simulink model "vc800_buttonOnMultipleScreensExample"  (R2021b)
settings: Solver=FixedStepDiscrete  StartTime=0.0  StopTime=10.0  FixedStep=0.01  RelTol=1e-3  EnableMultiTasking=on
PreLoadFcn:
  | try, model_open; catch, disp('Error occurred while executing model pre-load callback: model_open.m'); disp('Please assure that the MATLAB working directory is set to the model directory before opening.'); end
InitFcn:
  | try, model_open; catch, end
model workspace (MAT data in the model file):
  IOScreen_Label_XCoord = 1
  IOScreen_Row1_YCoord = 1
  IOScreen_Row2_YCoord = 12
  IOScreen_Value_XCoord = 110
  MainScreen_Row1_YCoord = 7
  MainScreen_Row2_YCoord = 23
  MainScreen_Symbols_XCoord = 1
  MainScreen_Units_XCoord = 69
  MainScreen_Value_XCoord = 64
undefined symbols (not defined in the file or in its folder): case, curr_screen, default, DISP, filtering, gesture, hex2dec, Mode, No, raptor_get_buildNum, raptor_get_safe_string, raptor_hwexp, raptor_xcp_function, Screens, VC800, Voltage
libraries: Raptor_display_lib x190, Raptor_lib x97, simulink_extras x11, Raptor_Datalogging_lib x10, simulink x2
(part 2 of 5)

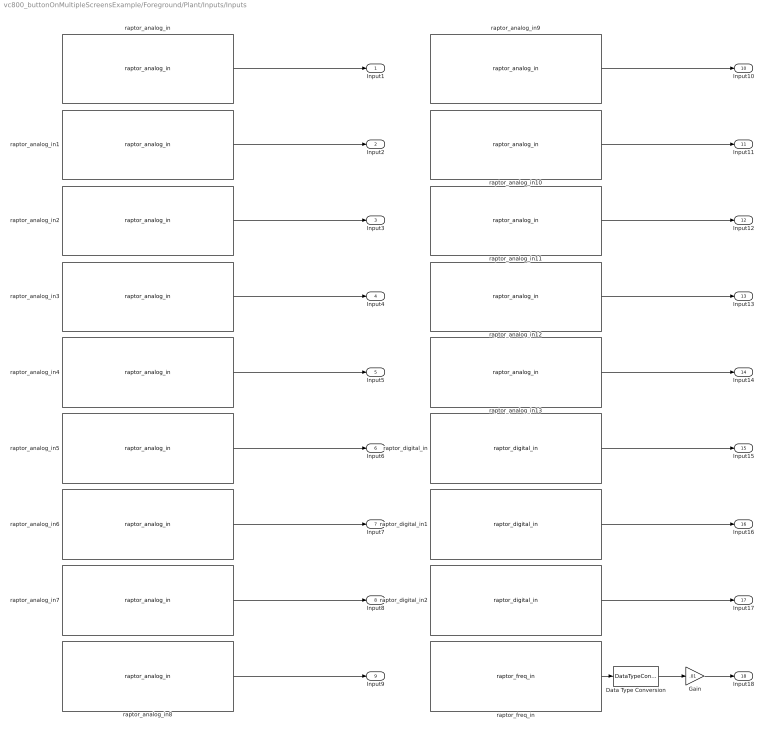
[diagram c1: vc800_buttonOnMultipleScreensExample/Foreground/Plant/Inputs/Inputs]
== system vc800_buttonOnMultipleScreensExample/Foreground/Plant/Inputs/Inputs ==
  Data Type Conversion : DataTypeConversion  OutDataTypeStr=single
  Gain : Gain  Gain=.01
  raptor_analog_in : Raptor_lib/Input & Output/raptor_analog_in  resourceValues=INPUT1|INPUT2|INPUT3|INPUT4|INPUT5|INPUT6|INPUT7|INPUT8|INPUT9|INPUT10|INPUT11|INPUT12|INPUT13|INPUT14|(None)  resource=INPUT1  rangeValues=Voltage Mode (0-10V)|Resistance Mode (0-500 Ohms)  range=Voltage Mode (0-10V)  filterrateValues=0.01 (~10 sec)|0.02|0.05|0.10 (Default)|0.25|0.50|0.75|1.00 (No filtering)  filterrate=1.00 (No filtering)  resolutionValues=[]  resolution=[]  pullUDValues=[]  pullUD=[]
  raptor_analog_in1 : Raptor_lib/Input & Output/raptor_analog_in  resourceValues=INPUT1|INPUT2|INPUT3|INPUT4|INPUT5|INPUT6|INPUT7|INPUT8|INPUT9|INPUT10|INPUT11|INPUT12|INPUT13|INPUT14|(None)  resource=INPUT2  rangeValues=Voltage Mode (0-10V)|Resistance Mode (0-500 Ohms)  range=Voltage Mode (0-10V)  filterrateValues=0.01 (~10 sec)|0.02|0.05|0.10 (Default)|0.25|0.50|0.75|1.00 (No filtering)  filterrate=1.00 (No filtering)  resolutionValues=[]  resolution=[]  pullUDValues=[]  pullUD=[]
  raptor_analog_in10 : Raptor_lib/Input & Output/raptor_analog_in  resourceValues=INPUT1|INPUT2|INPUT3|INPUT4|INPUT5|INPUT6|INPUT7|INPUT8|INPUT9|INPUT10|INPUT11|INPUT12|INPUT13|INPUT14|(None)  resource=INPUT11  rangeValues=Voltage Mode (0-10V)|Resistance Mode (0-500 Ohms)  range=Voltage Mode (0-10V)  filterrateValues=0.01 (~10 sec)|0.02|0.05|0.10 (Default)|0.25|0.50|0.75|1.00 (No filtering)  filterrate=1.00 (No filtering)  resolutionValues=[]  resolution=[]  pullUDValues=[]  pullUD=[]
  raptor_analog_in11 : Raptor_lib/Input & Output/raptor_analog_in  resourceValues=INPUT1|INPUT2|INPUT3|INPUT4|INPUT5|INPUT6|INPUT7|INPUT8|INPUT9|INPUT10|INPUT11|INPUT12|INPUT13|INPUT14|(None)  resource=INPUT12  rangeValues=Voltage Mode (0-10V)|Resistance Mode (0-500 Ohms)  range=Voltage Mode (0-10V)  filterrateValues=0.01 (~10 sec)|0.02|0.05|0.10 (Default)|0.25|0.50|0.75|1.00 (No filtering)  filterrate=1.00 (No filtering)  resolutionValues=[]  resolution=[]  pullUDValues=[]  pullUD=[]
  raptor_analog_in12 : Raptor_lib/Input & Output/raptor_analog_in  resourceValues=INPUT1|INPUT2|INPUT3|INPUT4|INPUT5|INPUT6|INPUT7|INPUT8|INPUT9|INPUT10|INPUT11|INPUT12|INPUT13|INPUT14|(None)  resource=INPUT13  rangeValues=Voltage Mode (0-10V)|Resistance Mode (0-500 Ohms)  range=Voltage Mode (0-10V)  filterrateValues=0.01 (~10 sec)|0.02|0.05|0.10 (Default)|0.25|0.50|0.75|1.00 (No filtering)  filterrate=1.00 (No filtering)  resolutionValues=[]  resolution=[]  pullUDValues=[]  pullUD=[]
  raptor_analog_in13 : Raptor_lib/Input & Output/raptor_analog_in  resourceValues=INPUT1|INPUT2|INPUT3|INPUT4|INPUT5|INPUT6|INPUT7|INPUT8|INPUT9|INPUT10|INPUT11|INPUT12|INPUT13|INPUT14|(None)  resource=INPUT14  rangeValues=Voltage Mode (0-10V)|Resistance Mode (0-500 Ohms)  range=Voltage Mode (0-10V)  filterrateValues=0.01 (~10 sec)|0.02|0.05|0.10 (Default)|0.25|0.50|0.75|1.00 (No filtering)  filterrate=1.00 (No filtering)  resolutionValues=[]  resolution=[]  pullUDValues=[]  pullUD=[]
  raptor_analog_in2 : Raptor_lib/Input & Output/raptor_analog_in  resourceValues=INPUT1|INPUT2|INPUT3|INPUT4|INPUT5|INPUT6|INPUT7|INPUT8|INPUT9|INPUT10|INPUT11|INPUT12|INPUT13|INPUT14|(None)  resource=INPUT3  rangeValues=Voltage Mode (0-10V)|Resistance Mode (0-500 Ohms)  range=Voltage Mode (0-10V)  filterrateValues=0.01 (~10 sec)|0.02|0.05|0.10 (Default)|0.25|0.50|0.75|1.00 (No filtering)  filterrate=1.00 (No filtering)  resolutionValues=[]  resolution=[]  pullUDValues=[]  pullUD=[]
  raptor_analog_in3 : Raptor_lib/Input & Output/raptor_analog_in  resourceValues=INPUT1|INPUT2|INPUT3|INPUT4|INPUT5|INPUT6|INPUT7|INPUT8|INPUT9|INPUT10|INPUT11|INPUT12|INPUT13|INPUT14|(None)  resource=INPUT4  rangeValues=Voltage Mode (0-10V)|Resistance Mode (0-500 Ohms)  range=Voltage Mode (0-10V)  filterrateValues=0.01 (~10 sec)|0.02|0.05|0.10 (Default)|0.25|0.50|0.75|1.00 (No filtering)  filterrate=1.00 (No filtering)  resolutionValues=[]  resolution=[]  pullUDValues=[]  pullUD=[]
  raptor_analog_in4 : Raptor_lib/Input & Output/raptor_analog_in  resourceValues=INPUT1|INPUT2|INPUT3|INPUT4|INPUT5|INPUT6|INPUT7|INPUT8|INPUT9|INPUT10|INPUT11|INPUT12|INPUT13|INPUT14|(None)  resource=INPUT5  rangeValues=Voltage Mode (0-10V)|Resistance Mode (0-500 Ohms)  range=Voltage Mode (0-10V)  filterrateValues=0.01 (~10 sec)|0.02|0.05|0.10 (Default)|0.25|0.50|0.75|1.00 (No filtering)  filterrate=1.00 (No filtering)  resolutionValues=[]  resolution=[]  pullUDValues=[]  pullUD=[]
  raptor_analog_in5 : Raptor_lib/Input & Output/raptor_analog_in  resourceValues=INPUT1|INPUT2|INPUT3|INPUT4|INPUT5|INPUT6|INPUT7|INPUT8|INPUT9|INPUT10|INPUT11|INPUT12|INPUT13|INPUT14|(None)  resource=INPUT6  rangeValues=Voltage Mode (0-10V)|Resistance Mode (0-500 Ohms)  range=Voltage Mode (0-10V)  filterrateValues=0.01 (~10 sec)|0.02|0.05|0.10 (Default)|0.25|0.50|0.75|1.00 (No filtering)  filterrate=1.00 (No filtering)  resolutionValues=[]  resolution=[]  pullUDValues=[]  pullUD=[]
  raptor_analog_in6 : Raptor_lib/Input & Output/raptor_analog_in  resourceValues=INPUT1|INPUT2|INPUT3|INPUT4|INPUT5|INPUT6|INPUT7|INPUT8|INPUT9|INPUT10|INPUT11|INPUT12|INPUT13|INPUT14|(None)  resource=INPUT7  rangeValues=Voltage Mode (0-10V)|Resistance Mode (0-500 Ohms)  range=Voltage Mode (0-10V)  filterrateValues=0.01 (~10 sec)|0.02|0.05|0.10 (Default)|0.25|0.50|0.75|1.00 (No filtering)  filterrate=1.00 (No filtering)  resolutionValues=[]  resolution=[]  pullUDValues=[]  pullUD=[]
  raptor_analog_in7 : Raptor_lib/Input & Output/raptor_analog_in  resourceValues=INPUT1|INPUT2|INPUT3|INPUT4|INPUT5|INPUT6|INPUT7|INPUT8|INPUT9|INPUT10|INPUT11|INPUT12|INPUT13|INPUT14|(None)  resource=INPUT8  rangeValues=Voltage Mode (0-10V)|Resistance Mode (0-500 Ohms)  range=Voltage Mode (0-10V)  filterrateValues=0.01 (~10 sec)|0.02|0.05|0.10 (Default)|0.25|0.50|0.75|1.00 (No filtering)  filterrate=1.00 (No filtering)  resolutionValues=[]  resolution=[]  pullUDValues=[]  pullUD=[]
  raptor_analog_in8 : Raptor_lib/Input & Output/raptor_analog_in  resourceValues=INPUT1|INPUT2|INPUT3|INPUT4|INPUT5|INPUT6|INPUT7|INPUT8|INPUT9|INPUT10|INPUT11|INPUT12|INPUT13|INPUT14|(None)  resource=INPUT9  rangeValues=Voltage Mode (0-10V)|Resistance Mode (0-500 Ohms)  range=Voltage Mode (0-10V)  filterrateValues=0.01 (~10 sec)|0.02|0.05|0.10 (Default)|0.25|0.50|0.75|1.00 (No filtering)  filterrate=1.00 (No filtering)  resolutionValues=[]  resolution=[]  pullUDValues=[]  pullUD=[]
  raptor_analog_in9 : Raptor_lib/Input & Output/raptor_analog_in  resourceValues=INPUT1|INPUT2|INPUT3|INPUT4|INPUT5|INPUT6|INPUT7|INPUT8|INPUT9|INPUT10|INPUT11|INPUT12|INPUT13|INPUT14|(None)  resource=INPUT10  rangeValues=Voltage Mode (0-10V)|Resistance Mode (0-500 Ohms)  range=Voltage Mode (0-10V)  filterrateValues=0.01 (~10 sec)|0.02|0.05|0.10 (Default)|0.25|0.50|0.75|1.00 (No filtering)  filterrate=1.00 (No filtering)  resolutionValues=[]  resolution=[]  pullUDValues=[]  pullUD=[]
  raptor_digital_in : Raptor_lib/Input & Output/raptor_digital_in  resourceValues=INPUT15|INPUT16|INPUT17|(None)  resource=INPUT15  pullUDValues=[]  pullUD=[]  upperThres='RAPTOR MASK DEFAULT'  lowerThres='RAPTOR MASK DEFAULT'
  raptor_digital_in1 : Raptor_lib/Input & Output/raptor_digital_in  resourceValues=INPUT15|INPUT16|INPUT17|(None)  resource=INPUT16  pullUDValues=[]  pullUD=[]  upperThres='RAPTOR MASK DEFAULT'  lowerThres='RAPTOR MASK DEFAULT'
  raptor_digital_in2 : Raptor_lib/Input & Output/raptor_digital_in  resourceValues=INPUT15|INPUT16|INPUT17|(None)  resource=INPUT17  pullUDValues=[]  pullUD=[]  upperThres='RAPTOR MASK DEFAULT'  lowerThres='RAPTOR MASK DEFAULT'
  raptor_freq_in : Raptor_lib/Input & Output/raptor_freq_in  minFreq=1  resourceValues=INPUT18|(None)  resource=INPUT18  pullUDValues=[]  pullUD=[]  interfaceValues=[]  interface=[]  hasDuty='RAPTOR MASK DEFAULT'  hasEdgeCount=off
  Input1 : Outport  VectorParamsAs1DForOutWhenUnconnected=off
  Input2 : Outport  Port=2  VectorParamsAs1DForOutWhenUnconnected=off
  Input3 : Outport  Port=3  VectorParamsAs1DForOutWhenUnconnected=off
  Input4 : Outport  Port=4  VectorParamsAs1DForOutWhenUnconnected=off
  Input5 : Outport  Port=5  VectorParamsAs1DForOutWhenUnconnected=off
  Input6 : Outport  Port=6  VectorParamsAs1DForOutWhenUnconnected=off
  Input7 : Outport  Port=7  VectorParamsAs1DForOutWhenUnconnected=off
  Input8 : Outport  Port=8  VectorParamsAs1DForOutWhenUnconnected=off
  Input9 : Outport  Port=9  VectorParamsAs1DForOutWhenUnconnected=off
  Input10 : Outport  Port=10  VectorParamsAs1DForOutWhenUnconnected=off
  Input11 : Outport  Port=11  VectorParamsAs1DForOutWhenUnconnected=off
  Input12 : Outport  Port=12  VectorParamsAs1DForOutWhenUnconnected=off
  Input13 : Outport  Port=13  VectorParamsAs1DForOutWhenUnconnected=off
  Input14 : Outport  Port=14  VectorParamsAs1DForOutWhenUnconnected=off
  Input15 : Outport  Port=15  VectorParamsAs1DForOutWhenUnconnected=off
  Input16 : Outport  Port=16  VectorParamsAs1DForOutWhenUnconnected=off
  Input17 : Outport  Port=17  VectorParamsAs1DForOutWhenUnconnected=off
  Input18 : Outport  Port=18  VectorParamsAs1DForOutWhenUnconnected=off
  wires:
  raptor_analog_in/1 -> Input1/1
  raptor_analog_in1/1 -> Input2/1
  raptor_analog_in2/1 -> Input3/1
  raptor_analog_in3/1 -> Input4/1
  raptor_analog_in4/1 -> Input5/1
  raptor_analog_in9/1 -> Input10/1
  raptor_analog_in8/1 -> Input9/1
  raptor_analog_in7/1 -> Input8/1
  raptor_analog_in6/1 -> Input7/1
  raptor_analog_in5/1 -> Input6/1
  raptor_analog_in12/1 -> Input13/1
  raptor_analog_in13/1 -> Input14/1
  raptor_analog_in11/1 -> Input12/1
  raptor_analog_in10/1 -> Input11/1
  raptor_digital_in/1 -> Input15/1
  raptor_digital_in2/1 -> Input17/1
  raptor_digital_in1/1 -> Input16/1
  raptor_freq_in/1 -> Data Type Conversion/1
  Gain/1 -> Input18/1
  Data Type Conversion/1 -> Gain/1

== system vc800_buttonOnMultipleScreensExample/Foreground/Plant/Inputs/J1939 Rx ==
  Process Illumination Message : Subsystem
  Process RPM Message : Subsystem
  raptor_can_rxmsg : Raptor_lib/CAN/raptor_can_rxmsg  canDefinition="struct('dbcFile', 'j1939_small.dbc','message', 'CL','comment', '','signals', {{'IlluminationBrightnessPercent'}},'enabled', [ 1;],'canBus', '''CAN1''','messageID', [ 416349696;],'idMask', [ 536870656;],'payloadMask', [],'payloadValue', [],'period', [ 0;],'mailbox', '''''','queueSize', [ 1;],'label', [ 0;],'ver', [ 2;],'showID', [ 0;],'showRaw', [ 0;],'fill', [ 0;],'editID', [ 1;],'signalOrder', [ 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"  canBus='CAN1'  mailbox=''  payloadMask=[]  payloadValue=[]  idMask=hex2dec('1FFFFF00')  queueSize=1  showID=0  label=0  fill=0  id=416349696  showRaw=0  showAge=1  signalOrder=1  signalInfo={{struct('Name', 'IlluminationBrightnessPercent','StartBit', [ 0;],'SignalSize', [ 8;],'ByteOrder', 'LittleEndian','ValueType', 'UNSIGNED','Class', 'uint8','Signed', [ 0;],'Factor', [ 0.4;],'Offset', [ 0;],'Min', [ 0;],'Max', [ 100;],'Units', '%','StartVal', [ 0;],'Comment', 'Commanded backlight brightness level for all cab displays','Multiplexed', [ 0;],'Multiplexor', [ 0;],'MultiplexMode_Min', [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  showRawMsg=0  useSimFunc=0  sim_func_name=''  useStartVals=0  extendedId=1
  raptor_can_rxmsg1 : Raptor_lib/CAN/raptor_can_rxmsg  canDefinition=struct('dbcFile', 'j1939_small.dbc','message', 'EEC1','comment', '','signals', {{'EngSpeed'}},'enabled', [ 1;],'canBus', '''CAN1''','messageID', [ 217056256;],'idMask', [ 536870656;],'payloadMask', [],'payloadValue', [],'period', [ 0;],'mailbox', '''''','queueSize', [ 1;],'label', [ 0;],'ver', [ 2;],'showID', [ 0;],'showRaw', [ 0;],'fill', [ 0;],'editID', [ 1;],'signalOrder', [ 1;])  canBus='CAN1'  mailbox=''  payloadMask=[]  payloadValue=[]  idMask=hex2dec('1FFFFF00')  queueSize=1  showID=0  label=0  fill=0  id=217056256  showRaw=0  showAge=1  signalOrder=1  signalInfo={{struct('Name', 'EngSpeed','StartBit', [ 24;],'SignalSize', [ 16;],'ByteOrder', 'LittleEndian','ValueType', 'UNSIGNED','Class', 'uint16','Signed', [ 0;],'Factor', [ 0.125;],'Offset', [ 0;],'Min', [ 0;],'Max', [ 8031.88;],'Units', 'rpm','StartVal', [ 0;],'Comment', 'Actual engine speed which is calculated over a minimum crankshaft angle of 720 degrees divided by the number of cylinders.','Multiple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  showRawMsg=0  useSimFunc=0  sim_func_name=''  useStartVals=0  extendedId=1
  Engine RPM : Outport  VectorParamsAs1DForOutWhenUnconnected=off
  Engine RPM Valid : Outport  Port=2  VectorParamsAs1DForOutWhenUnconnected=off
  Illumination : Outport  Port=3  VectorParamsAs1DForOutWhenUnconnected=off
  Illumination1 : Outport  Port=4  VectorParamsAs1DForOutWhenUnconnected=off
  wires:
  Process RPM Message/1(EngineRPM) -> Engine RPM/1
  Process Illumination Message/1(Illumination) -> Illumination/1
  Process RPM Message/2(EngineRPMValid) -> Engine RPM Valid/1
  raptor_can_rxmsg1/1 -> Process RPM Message/1(AgeCount)
  raptor_can_rxmsg1/2 -> Process RPM Message/2(Data)
  raptor_can_rxmsg/1 -> Process Illumination Message/1(AgeCount)
  raptor_can_rxmsg/2 -> Process Illumination Message/2(Data)
  Process Illumination Message/2(IlluminationValid) -> Illumination1/1

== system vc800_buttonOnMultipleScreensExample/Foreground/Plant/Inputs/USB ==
  raptor_fileIO_USBStatus : Raptor_Datalogging_lib/raptor_fileIO_USBStatus  showInserted=on  showEjectReady=on  showPath=on  showReadyToLog=on
  raptor_fileIO_getFreeSpace : Raptor_Datalogging_lib/raptor_fileIO_getFreeSpace  resourceValues=USB|(None)  resource=USB
  raptor_string : Raptor_lib/Strings/raptor_string  stringName=''  string=''  dynamicSize=Fixed Size  strSize=20  storage=Volatile (RAM)  calVisible=off  calAccess=4  strFunction=raptor_xcp_function(gcb)
  USBInserted : Outport  VectorParamsAs1DForOutWhenUnconnected=off
  USBEjectReady : Outport  Port=2  VectorParamsAs1DForOutWhenUnconnected=off
  USBPath : Outport  Port=3  VectorParamsAs1DForOutWhenUnconnected=off
  USBReadyToLog : Outport  Port=4  VectorParamsAs1DForOutWhenUnconnected=off
  USBFreeSpace : Outport  Port=5  VectorParamsAs1DForOutWhenUnconnected=off
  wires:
  raptor_fileIO_USBStatus/1 -> USBInserted/1
  raptor_fileIO_USBStatus/4 -> USBReadyToLog/1
  raptor_fileIO_USBStatus/3 -> USBPath/1
  raptor_fileIO_USBStatus/2 -> USBEjectReady/1
  raptor_string/1 -> raptor_fileIO_USBStatus/1
  raptor_fileIO_getFreeSpace/1 -> USBFreeSpace/1

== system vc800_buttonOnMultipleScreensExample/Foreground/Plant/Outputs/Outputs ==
  Output1 : Inport
  Output2 : Inport  Port=2
  Output3 : Inport  Port=3
  Output4 : Inport  Port=4
  Output5 : Inport  Port=5
  Output6 : Inport  Port=6
  Output7 : Inport  Port=7
  Output8 : Inport  Port=8
  raptor_digital_out : Raptor_lib/Input & Output/raptor_digital_out  resourceValues=OUTPUT1|OUTPUT2|OUTPUT3|OUTPUT4|BUZZER_MUTE|BUZZER|OUTPUT5|OUTPUT6|OUTPUT7|OUTPUT8|(None)  resource=OUTPUT1  driverTypeValues=Low Side  driverType=Low Side
  raptor_digital_out1 : Raptor_lib/Input & Output/raptor_digital_out  resourceValues=OUTPUT1|OUTPUT2|OUTPUT3|OUTPUT4|BUZZER_MUTE|BUZZER|OUTPUT5|OUTPUT6|OUTPUT7|OUTPUT8|(None)  resource=OUTPUT2  driverTypeValues=Low Side  driverType=Low Side
  raptor_digital_out2 : Raptor_lib/Input & Output/raptor_digital_out  resourceValues=OUTPUT1|OUTPUT2|OUTPUT3|OUTPUT4|BUZZER_MUTE|BUZZER|OUTPUT5|OUTPUT6|OUTPUT7|OUTPUT8|(None)  resource=OUTPUT3  driverTypeValues=Low Side  driverType=Low Side
  raptor_digital_out3 : Raptor_lib/Input & Output/raptor_digital_out  resourceValues=OUTPUT1|OUTPUT2|OUTPUT3|OUTPUT4|BUZZER_MUTE|BUZZER|OUTPUT5|OUTPUT6|OUTPUT7|OUTPUT8|(None)  resource=OUTPUT4  driverTypeValues=Low Side  driverType=Low Side
  raptor_digital_out4 : Raptor_lib/Input & Output/raptor_digital_out  resourceValues=OUTPUT1|OUTPUT2|OUTPUT3|OUTPUT4|BUZZER_MUTE|BUZZER|OUTPUT5|OUTPUT6|OUTPUT7|OUTPUT8|(None)  resource=OUTPUT5  driverTypeValues=Low Side  driverType=Low Side
  raptor_digital_out5 : Raptor_lib/Input & Output/raptor_digital_out  resourceValues=OUTPUT1|OUTPUT2|OUTPUT3|OUTPUT4|BUZZER_MUTE|BUZZER|OUTPUT5|OUTPUT6|OUTPUT7|OUTPUT8|(None)  resource=OUTPUT6  driverTypeValues=Low Side  driverType=Low Side
  raptor_digital_out6 : Raptor_lib/Input & Output/raptor_digital_out  resourceValues=OUTPUT1|OUTPUT2|OUTPUT3|OUTPUT4|BUZZER_MUTE|BUZZER|OUTPUT5|OUTPUT6|OUTPUT7|OUTPUT8|(None)  resource=OUTPUT7  driverTypeValues=Low Side  driverType=Low Side
  raptor_digital_out7 : Raptor_lib/Input & Output/raptor_digital_out  resourceValues=OUTPUT1|OUTPUT2|OUTPUT3|OUTPUT4|BUZZER_MUTE|BUZZER|OUTPUT5|OUTPUT6|OUTPUT7|OUTPUT8|(None)  resource=OUTPUT8  driverTypeValues=Low Side  driverType=Low Side
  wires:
  Output1/1 -> raptor_digital_out/1
  Output2/1 -> raptor_digital_out1/1
  Output4/1 -> raptor_digital_out3/1
  Output3/1 -> raptor_digital_out2/1
  Output7/1 -> raptor_digital_out6/1
  Output6/1 -> raptor_digital_out5/1
  Output5/1 -> raptor_digital_out4/1
  Output8/1 -> raptor_digital_out7/1

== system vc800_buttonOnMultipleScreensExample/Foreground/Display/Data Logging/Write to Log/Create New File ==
  Path : Inport
  Action Port : ActionPort  ActionPortLabel=else
  raptor_fileIO_open1 : Raptor_Datalogging_lib/raptor_fileIO_open  resourceValues=USB|(None)  resource=USB  modeValues=Read Only|Write Only - Overwrite|Read/Write - Update|Read/Write - Overwrite  mode=2
  Handle : Outport  VectorParamsAs1DForOutWhenUnconnected=off
  Success : Outport  Port=2  VectorParamsAs1DForOutWhenUnconnected=off
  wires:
  Path/1 -> raptor_fileIO_open1/1
  raptor_fileIO_open1/1 -> Handle/1
  raptor_fileIO_open1/2 -> Success/1

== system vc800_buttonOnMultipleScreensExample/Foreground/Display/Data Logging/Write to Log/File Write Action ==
  In Bus Element{2..5} (4 alike) : Inport
  In2 : Inport  Port=2
  Enable : EnablePort
  Add : Sum
  Constant : Constant  OutDataTypeStr=uint32
  Counter Limited : simulink/Sources/Counter Limited  uplimit=65535  tsamp=-1
  Data Type Conversion1 : DataTypeConversion
  Data Type Conversion10 : DataTypeConversion
  Data Type Conversion2 : DataTypeConversion
  Sync File : Subsystem  TreatAsAtomicUnit=on
  Sync every 10 Seconds : Subsystem
  Terminator1 : Terminator
  raptor_data_def : Raptor_lib/Data Storage/raptor_data_def  dataName='LogCounter'  initValue=0  dataType=uint32  storage=Volatile (RAM)  calVisible=on  calType=Measurement  calDispType=Number  calEnum={'False', 'True'}  calGain=1.0  calOffset=0  calMin=-inf  calMax=inf  calFormat='-1'  calUnit=''  calHelp=''  calAccess=1  calFunction=raptor_xcp_function(gcb)  calDispHeaders=off  calColHeaders={'Col1' 'Col2' 'Col3'}  calRowHeaders={'Row1' 'Row2' 'Row3'}
  raptor_data_read1 : Raptor_lib/Data Storage/raptor_data_read  dataName='LogCounter'  dataShape=Scalar  idxSource=Input  idxRow=1  idxCol=1
  raptor_data_write : Raptor_lib/Data Storage/raptor_data_write  dataName='LogCounter'  dataShape=Scalar  idxSource=Input Port  idxRow=1  idxCol=1
  raptor_fileIO_close : Raptor_Datalogging_lib/raptor_fileIO_close  resourceValues=USB|(None)  resource=USB
  raptor_fileIO_write : Raptor_Datalogging_lib/raptor_fileIO_write  resourceValues=Data|USB|(None)  resource=USB
  raptor_string : Raptor_lib/Strings/raptor_string  stringName=''  string=''  dynamicSize=Fixed Size  strSize=100  storage=Volatile (RAM)  calVisible=on  calAccess=4  strFunction=raptor_xcp_function(gcb)
  raptor_string_length : Raptor_lib/Strings/raptor_string_length  outSize=10
  raptor_string_printf1 : Raptor_lib/Strings/raptor_string_printf  formatString=' %u %u %f %u %f %.8u\n'
  raptor_string_toArray : Raptor_lib/Strings/raptor_string_toArray  outSize=100
  raptor_time1 : Raptor_lib/Triggers/raptor_time  unit=milliseconds
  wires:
  Sync every 10 Seconds/1(TimeToSync) -> Sync File/Enable
  raptor_string_toArray/1 -> raptor_fileIO_write/2
  raptor_string_printf1/1 -> raptor_string_toArray/1, raptor_string_length/1
  raptor_string/1 -> raptor_string_printf1/1
  raptor_string_length/1 -> raptor_fileIO_write/3
  Data Type Conversion10/1 -> raptor_string_printf1/2
  raptor_fileIO_write/2 -> Terminator1/1
  raptor_fileIO_write/1 -> raptor_fileIO_close/1
  In2/1 -> raptor_fileIO_write/1, Sync File/1(In1)
  Constant/1 -> Add/2
  Add/1 -> raptor_data_write/1
  raptor_data_read1/1 -> Add/1
  Counter Limited/1 -> Data Type Conversion10/1
  raptor_time1/1 -> raptor_string_printf1/7
  In Bus Element5/1 -> Data Type Conversion2/1
  In Bus Element4/1 -> raptor_string_printf1/6
  In Bus Element3/1 -> Data Type Conversion1/1
  In Bus Element2/1 -> raptor_string_printf1/4
  Data Type Conversion1/1 -> raptor_string_printf1/3
  Data Type Conversion2/1 -> raptor_string_printf1/5

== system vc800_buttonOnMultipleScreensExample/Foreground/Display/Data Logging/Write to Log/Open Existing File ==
  Path : Inport
  Action Port : ActionPort  ActionPortLabel=if(u1)
  File Seek : Subsystem
  Merge : Subsystem
  raptor_fileIO_open1 : Raptor_Datalogging_lib/raptor_fileIO_open  resourceValues=Data|USB|(None)  resource=USB  modeValues=Read Only|Write Only - Overwrite|Read/Write - Update|Read/Write - Overwrite  mode=3
  Handle : Outport  VectorParamsAs1DForOutWhenUnconnected=off
  Sucess : Outport  Port=2  VectorParamsAs1DForOutWhenUnconnected=off
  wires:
  Path/1 -> raptor_fileIO_open1/1
  Merge/1(Handle) -> Handle/1
  Merge/2(Success) -> Sucess/1
  raptor_fileIO_open1/1 -> File Seek/1(Open File Handle)
  raptor_fileIO_open1/2 -> File Seek/2(Open Success)
  File Seek/1(Seek File Handle Success) -> Merge/1(File Handle Success)
  File Seek/2(Seek Success) -> Merge/2(File Open Success)
  File Seek/3(Seek File Handle Failure) -> Merge/3(File Handle Failure)
  File Seek/4(Seek Failure) -> Merge/4(File Open Failure)

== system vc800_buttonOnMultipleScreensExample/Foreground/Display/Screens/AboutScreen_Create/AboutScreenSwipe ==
  note: This function is called when a swipe action occurs. The gesture input will provide the gesture detected: 0 = UP 1 = DOWN 2 = LEFT 3 = RIGHT
  AboutScreenSwipe : TriggerPort  TriggerType=function-call  IsSimulinkFunction=on  FunctionName=AboutScreenSwipe  FunctionVisibility=scoped  VariantControl=Variant  PortDimensions=1
  Constant : Constant  Value=5  OutDataTypeStr=uint8
  Function Caller : FunctionCaller  FunctionPrototype=Screens.Navigation(gesture,curr_screen)  InputArgumentSpecifications=<Enter example>  OutputArgumentSpecifications=<Enter example>
  gesture : ArgIn  OutDataTypeStr=uint8  ArgumentName=gesture
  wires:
  Constant/1 -> Function Caller/2
  gesture/1 -> Function Caller/1

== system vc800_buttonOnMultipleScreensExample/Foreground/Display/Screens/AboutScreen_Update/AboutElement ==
  function : TriggerPort  TriggerType=function-call  VariantControl=Variant
  Add{,2..4} (4 alike) : Sum
  Constant{1,3,5..6,8} (5 alike) : Constant  Value=400  OutDataTypeStr=int32
  Constant2 : Constant  Value=30  OutDataTypeStr=int32
  Constant7 : Constant  Value=100  OutDataTypeStr=int32
  display_draw_text1 : Raptor_display_lib/Drawing Functions/display_draw_text  textPort=off  textVal='Raptor Version : '  colorPort=off  col=FFFF  opacity=100  font=Future  fontFile=''  heightPort=off  height=20  hAlign=Right  vAlign=Top  spacing=0  layer=Background  pnPort=off
  display_draw_text10 : Raptor_display_lib/Drawing Functions/display_draw_text  textPort=off  textVal=get_param(bdroot, 'ModelVersion')  colorPort=off  col=FFFF  opacity=100  font=Future  fontFile=''  heightPort=off  height=20  hAlign=Left  vAlign=Top  spacing=0  layer=Background  pnPort=off
  display_draw_text11 : Raptor_display_lib/Drawing Functions/display_draw_text  textPort=off  textVal='Build Number : '  colorPort=off  col=FFFF  opacity=100  font=Future  fontFile=''  heightPort=off  height=20  hAlign=Right  vAlign=Top  spacing=0  layer=Background  pnPort=off
  display_draw_text12 : Raptor_display_lib/Drawing Functions/display_draw_text  textPort=off  textVal=num2str(raptor_get_buildNum(bdroot(gcb)))  colorPort=off  col=FFFF  opacity=100  font=Future  fontFile=''  heightPort=off  height=20  hAlign=Left  vAlign=Top  spacing=0  layer=Background  pnPort=off
  display_draw_text2 : Raptor_display_lib/Drawing Functions/display_draw_text  textPort=off  textVal='MATLAB Version : '  colorPort=off  col=FFFF  opacity=100  font=Future  fontFile=''  heightPort=off  height=20  hAlign=Right  vAlign=Top  spacing=0  layer=Background  pnPort=off
  display_draw_text3 : Raptor_display_lib/Drawing Functions/display_draw_text  textPort=off  textVal=version  colorPort=off  col=FFFF  opacity=100  font=Future  fontFile=''  heightPort=off  height=20  hAlign=Left  vAlign=Top  spacing=0  layer=Background  pnPort=off
  display_draw_text6 : Raptor_display_lib/Drawing Functions/display_draw_text  textPort=off  textVal=raptor_hwexp('COMMAND:RAPTOR_VERSION')  colorPort=off  col=FFFF  opacity=100  font=Future  fontFile=''  heightPort=off  height=20  hAlign=Left  vAlign=Top  spacing=0  layer=Background  pnPort=off
  display_draw_text7 : Raptor_display_lib/Drawing Functions/display_draw_text  textPort=off  textVal='Application Name : '  colorPort=off  col=FFFF  opacity=100  font=Future  fontFile=''  heightPort=off  height=20  hAlign=Right  vAlign=Top  spacing=0  layer=Background  pnPort=off
  display_draw_text8 : Raptor_display_lib/Drawing Functions/display_draw_text  textPort=off  textVal=bdroot  colorPort=off  col=FFFF  opacity=100  font=Future  fontFile=''  heightPort=off  height=20  hAlign=Left  vAlign=Top  spacing=0  layer=Background  pnPort=off
  display_draw_text9 : Raptor_display_lib/Drawing Functions/display_draw_text  textPort=off  textVal='Model Version : '  colorPort=off  col=FFFF  opacity=100  font=Future  fontFile=''  heightPort=off  height=20  hAlign=Right  vAlign=Top  spacing=0  layer=Background  pnPort=off
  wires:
  Constant1/1 -> display_draw_text6/1, display_draw_text1/1
  Add/1 -> display_draw_text2/2, display_draw_text3/2
  Constant3/1 -> display_draw_text2/1, display_draw_text3/1
  Constant5/1 -> display_draw_text7/1, display_draw_text8/1
  Add2/1 -> Add/1, display_draw_text6/2, display_draw_text1/2
  Constant2/1 -> Add3/2, Add4/2, Add2/2, Add/2
  Add4/1 -> Add2/1, display_draw_text11/2, display_draw_text12/2
  Constant8/1 -> display_draw_text11/1, display_draw_text12/1
  Add3/1 -> Add4/1, display_draw_text9/2, display_draw_text10/2
  Constant6/1 -> display_draw_text9/1, display_draw_text10/1
  Constant7/1 -> display_draw_text7/2, display_draw_text8/2, Add3/1

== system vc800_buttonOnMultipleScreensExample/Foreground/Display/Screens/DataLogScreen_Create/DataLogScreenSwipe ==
  note: This function is called when a swipe action occurs. The gesture input will provide the gesture detected: 0 = UP 1 = DOWN 2 = LEFT 3 = RIGHT
  DataLogScreenSwipe : TriggerPort  TriggerType=function-call  IsSimulinkFunction=on  FunctionName=DataLogScreenSwipe  FunctionVisibility=scoped  VariantControl=Variant  PortDimensions=1
  Constant : Constant  Value=4  OutDataTypeStr=uint8
  Function Caller : FunctionCaller  FunctionPrototype=Screens.Navigation(gesture,curr_screen)  InputArgumentSpecifications=<Enter example>  OutputArgumentSpecifications=<Enter example>
  gesture : ArgIn  OutDataTypeStr=uint8  ArgumentName=gesture
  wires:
  gesture/1 -> Function Caller/1
  Constant/1 -> Function Caller/2

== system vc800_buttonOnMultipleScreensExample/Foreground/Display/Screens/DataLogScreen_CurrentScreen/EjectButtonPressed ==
  Trigger : TriggerPort  TriggerType=falling  VariantControl=Variant  PortDimensions=1
  raptor_fileIO_USBEject : Raptor_Datalogging_lib/raptor_fileIO_USBEject  variable=0

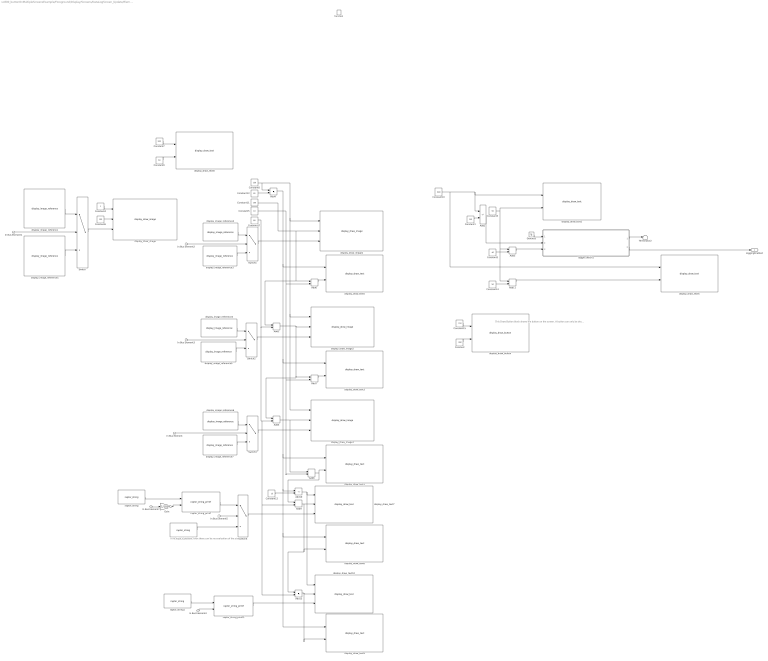
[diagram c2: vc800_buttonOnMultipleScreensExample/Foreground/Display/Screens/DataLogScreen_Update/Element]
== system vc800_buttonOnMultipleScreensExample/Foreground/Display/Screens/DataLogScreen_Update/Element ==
  note: If no drive is present, then there can be no evaluation of the size
  note: This Draw Button block shows the button on the screen. A button can only be drawn once per screen.
  In Bus Element{,1..5} (6 alike) : Inport
  In Bus Element7 : Inport  Port=2
  function : TriggerPort  TriggerType=function-call  VariantControl=Variant
  Add{1,3..9,11,13} (10 alike) : Sum
  Add10 : Sum  Inputs=+-
  Add2 : Sum  Inputs=+-
  Constant : Constant  Value=390  OutDataTypeStr=Inherit: Inherit via back propagation
  Constant1 : Constant  Value=140  OutDataTypeStr=int32
  Constant10 : Constant  Value=600  OutDataTypeStr=int32
  Constant11 : Constant  Value=100  OutDataTypeStr=int32
  Constant12 : Constant  Value=15  OutDataTypeStr=int32
  Constant13 : Constant  Value=65  OutDataTypeStr=int32
  Constant14 : Constant  Value=50  OutDataTypeStr=int32
  Constant15 : Constant  Value=720  OutDataTypeStr=Inherit: Inherit via back propagation
  Constant17 : Constant  Value=60  OutDataTypeStr=int32
  Constant2 : Constant  Value=40  OutDataTypeStr=int32
  Constant3 : Constant  Value=50  OutDataTypeStr=int32
  Constant4 : Constant  OutDataTypeStr=int32
  Constant5 : Constant  Value=19  OutDataTypeStr=int32
  Constant6 : Constant  Value=100  OutDataTypeStr=int32
  Constant7 : Constant  Value=200  OutDataTypeStr=int32
  Constant8 : Constant  Value=150  OutDataTypeStr=int32
  Constant9 : Constant  Value=50  OutDataTypeStr=int32
  Gain : Gain  Gain=1/1024  OutDataTypeStr=uint32
  Ground3 : Ground
  Switch{,1..4} (5 alike) : Switch  Criteria=u2 ~= 0
  Terminator2 : Terminator
  Toggle Switch1 : Subsystem  mask(Display Toggle){InitialCondition=0}
      mask prompts: InitialCondition "Initial Condition"
      mask help: Draws a toggle switch onto the screen that will hold either an off or an on state
  display_draw_button : Raptor_display_lib/Drawing Functions/display_draw_button  ButtonName='GoToAbout'
  display_draw_image{,1..3} (4 alike) : Raptor_display_lib/Drawing Functions/display_draw_image  imagePort=on  imageFile=USB_Icon_Sprite_Green_25perc.png  opacityPort=off  opacity=100  drawMode=Draw Entire Image  alpha=Draw as Transparent  layer=Background  drawModeXY=Top Left  pnPort=off
  display_draw_text1 : Raptor_display_lib/Drawing Functions/display_draw_text  textPort=off  textVal='Ready to Eject'  colorPort=off  col=FFFF  opacity=100  font=Future  fontFile=''  heightPort=off  height=20  hAlign=Left  vAlign=Top  spacing=0  layer=Background  pnPort=off
  display_draw_text10 : Raptor_display_lib/Drawing Functions/display_draw_text  textPort=on  textVal='Eject Ready'  colorPort=off  col=FFFF  opacity=100  font=Future  fontFile=''  heightPort=off  height=20  hAlign=Right  vAlign=Top  spacing=0  layer=Background  pnPort=off
  display_draw_text2 : Raptor_display_lib/Drawing Functions/display_draw_text  textPort=off  textVal='Control'  colorPort=off  col=FFFF  opacity=100  font=Future  fontFile=''  heightPort=off  height=30  hAlign=Center  vAlign=Top  spacing=0  layer=Background  pnPort=off
  display_draw_text3 : Raptor_display_lib/Drawing Functions/display_draw_text  textPort=off  textVal='Logging Active'  colorPort=off  col=FFFF  opacity=100  font=Future  fontFile=''  heightPort=off  height=20  hAlign=Left  vAlign=Top  spacing=0  layer=Background  pnPort=off
  display_draw_text4 : Raptor_display_lib/Drawing Functions/display_draw_text  textPort=off  textVal='Logging'  colorPort=off  col=FFFF  opacity=100  font=Future  fontFile=''  heightPort=off  height=20  hAlign=Left  vAlign=Top  spacing=0  layer=Background  pnPort=off
  display_draw_text5 : Raptor_display_lib/Drawing Functions/display_draw_text  textPort=off  textVal='Ready to Log'  colorPort=off  col=FFFF  opacity=100  font=Future  fontFile=''  heightPort=off  height=20  hAlign=Left  vAlign=Top  spacing=0  layer=Background  pnPort=off
  display_draw_text6 : Raptor_display_lib/Drawing Functions/display_draw_text  textPort=off  textVal='USB Free Space'  colorPort=off  col=FFFF  opacity=100  font=Future  fontFile=''  heightPort=off  height=20  hAlign=Left  vAlign=Top  spacing=0  layer=Background  pnPort=off
  display_draw_text7 : Raptor_display_lib/Drawing Functions/display_draw_text  textPort=on  textVal='Eject Ready'  colorPort=off  col=FFFF  opacity=100  font=Future  fontFile=''  heightPort=off  height=20  hAlign=Right  vAlign=Top  spacing=0  layer=Background  pnPort=off
  display_draw_text8 : Raptor_display_lib/Drawing Functions/display_draw_text  textPort=off  textVal='Status'  colorPort=off  col=FFFF  opacity=100  font=Future  fontFile=''  heightPort=off  height=30  hAlign=Center  vAlign=Top  spacing=0  layer=Background  pnPort=off
  display_draw_text9 : Raptor_display_lib/Drawing Functions/display_draw_text  textPort=off  textVal='# Lines Logged'  colorPort=off  col=FFFF  opacity=100  font=Future  fontFile=''  heightPort=off  height=20  hAlign=Left  vAlign=Top  spacing=0  layer=Background  pnPort=off
  display_image_reference : Raptor_display_lib/Drawing Functions/display_image_reference  imageFile=USB_Icon_Sprite_Green_25perc.png
  display_image_reference1 : Raptor_display_lib/Drawing Functions/display_image_reference  imageFile=USB_Icon_Sprite_Red_25perc.png
  display_image_reference2 : Raptor_display_lib/Drawing Functions/display_image_reference  imageFile=Oval Driver@2x.png
  display_image_reference3 : Raptor_display_lib/Drawing Functions/display_image_reference  imageFile=Oval Active@2x.png
  display_image_reference4 : Raptor_display_lib/Drawing Functions/display_image_reference  imageFile=Oval Driver@2x.png
  display_image_reference5 : Raptor_display_lib/Drawing Functions/display_image_reference  imageFile=Oval Active@2x.png
  display_image_reference6 : Raptor_display_lib/Drawing Functions/display_image_reference  imageFile=Oval Driver@2x.png
  display_image_reference7 : Raptor_display_lib/Drawing Functions/display_image_reference  imageFile=Oval Active@2x.png
  raptor_string : Raptor_lib/Strings/raptor_string  stringName=''  string=''  dynamicSize=Fixed Size  strSize=20  storage=Volatile (RAM)  calVisible=off  calAccess=4  strFunction=raptor_xcp_function(gcb)
  raptor_string1 : Raptor_lib/Strings/raptor_string  stringName=''  string=''  dynamicSize=Fixed Size  strSize=20  storage=Volatile (RAM)  calVisible=off  calAccess=4  strFunction=raptor_xcp_function(gcb)
  raptor_string2 : Raptor_lib/Strings/raptor_string  stringName=''  string='N/A'  dynamicSize=Size from initial value  strSize=20  storage=Volatile (RAM)  calVisible=off  calAccess=4  strFunction=raptor_xcp_function(gcb)
  raptor_string_printf : Raptor_lib/Strings/raptor_string_printf  formatString='%u KB'
  raptor_string_printf1 : Raptor_lib/Strings/raptor_string_printf  formatString='%u'
  LoggingEnabled : Outport  VectorParamsAs1DForOutWhenUnconnected=off
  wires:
  Constant2/1 -> Add3/2
  Add2/1 -> Toggle Switch1/2(x)
  Toggle Switch1/1(next) -> Terminator2/1
  Toggle Switch1/2(out) -> LoggingEnabled/1
  Ground3/1 -> Toggle Switch1/1(prev)
  Constant10/1 -> display_draw_text4/1, Add2/1, display_draw_text2/1
  Constant1/1 -> Add2/2
  Add3/1 -> Toggle Switch1/3(y)
  Constant6/1 -> display_draw_image/2
  Constant4/1 -> display_draw_image/1
  display_image_reference/1 -> Switch/1
  display_image_reference1/1 -> Switch/3
  In Bus Element1/1 -> Switch/2
  Switch/1 -> display_draw_image/3
  Switch1/1 -> display_draw_image1/3
  Constant8/1 -> Add4/1, display_draw_image3/1, display_draw_image2/1, display_draw_image1/1
  Constant11/1 -> Add1/1, Add6/1, display_draw_image1/2
  Add1/1 -> Add7/1, Add5/1, display_draw_image2/2
  Switch2/1 -> display_draw_image2/3
  Switch3/1 -> display_draw_image3/3
  display_image_reference7/1 -> Switch3/3
  display_image_reference6/1 -> Switch3/1
  In Bus Element/1 -> Switch3/2
  Constant13/1 -> Add4/2
  Constant17/1 -> Add13/2, Add9/2, Add5/2, Add1/2
  Add5/1 -> Add8/1, display_draw_image3/2
  Constant5/1 -> Add8/2, Add7/2, Add6/2
  Add6/1 -> display_draw_text5/2
  Add7/1 -> display_draw_text3/2
  Add8/1 -> Add9/1, display_draw_text1/2
  raptor_string/1 -> raptor_string_printf/1
  In Bus Element7/1 -> Gain/1
  Constant7/1 -> display_draw_text8/1
  Constant9/1 -> display_draw_text8/2
  Constant12/1 -> Add10/2
  Constant3/1 -> Add11/1, Add3/1, display_draw_text2/2
  Add10/1 -> display_draw_text10/1, display_draw_text7/1
  Add13/1 -> display_draw_text10/2, display_draw_text9/2
  raptor_string_printf1/1 -> display_draw_text10/3
  In Bus Element4/1 -> raptor_string_printf1/2
  raptor_string1/1 -> raptor_string_printf1/1
  Add9/1 -> Add13/1, display_draw_text6/2, display_draw_text7/2
  Add4/1 -> display_draw_text5/1, Add10/1, display_draw_text9/1, display_draw_text6/1, display_draw_text1/1, display_draw_text3/1
  raptor_string_printf/1 -> Switch4/1
  Switch4/1 -> display_draw_text7/3
  raptor_string2/1 -> Switch4/3
  In Bus Element5/1 -> Switch4/2
  Gain/1 -> raptor_string_printf/2
  In Bus Element3/1 -> Switch2/2
  display_image_reference4/1 -> Switch2/1
  display_image_reference5/1 -> Switch2/3
  display_image_reference3/1 -> Switch1/3
  display_image_reference2/1 -> Switch1/1
  In Bus Element2/1 -> Switch1/2
  Add11/1 -> display_draw_text4/2
  Constant14/1 -> Add11/2
  Constant15/1 -> display_draw_button/1
  Constant/1 -> display_draw_button/2

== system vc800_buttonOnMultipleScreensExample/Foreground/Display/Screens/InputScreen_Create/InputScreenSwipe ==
  note: This function is called when a swipe action occurs. The gesture input will provide the gesture detected: 0 = UP 1 = DOWN 2 = LEFT 3 = RIGHT
  InputScreenSwipe : TriggerPort  TriggerType=function-call  IsSimulinkFunction=on  FunctionName=InputScreenSwipe  FunctionVisibility=scoped  VariantControl=Variant  PortDimensions=1
  Constant : Constant  Value=2  OutDataTypeStr=uint8
  Function Caller : FunctionCaller  FunctionPrototype=Screens.Navigation(gesture,curr_screen)  InputArgumentSpecifications=<Enter example>  OutputArgumentSpecifications=<Enter example>
  gesture : ArgIn  OutDataTypeStr=uint8  ArgumentName=gesture
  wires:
  Constant/1 -> Function Caller/2
  gesture/1 -> Function Caller/1

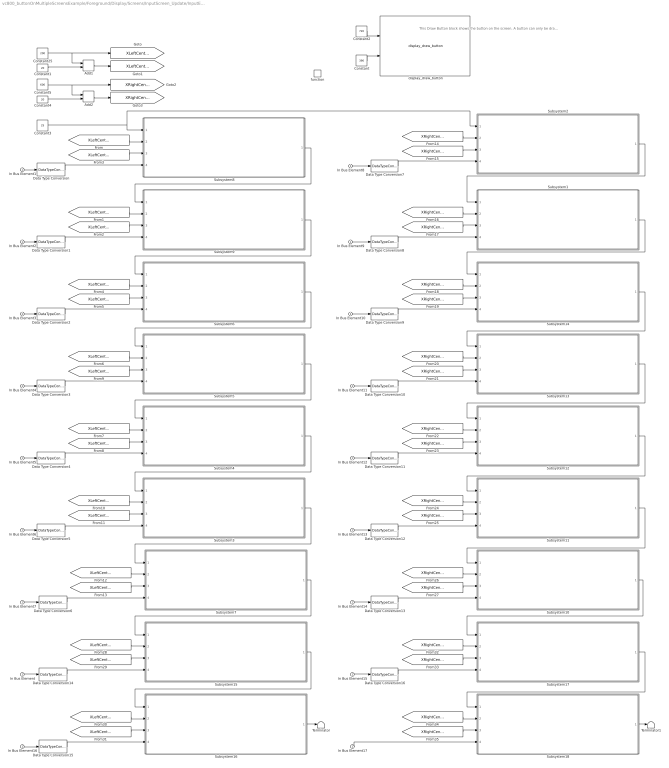
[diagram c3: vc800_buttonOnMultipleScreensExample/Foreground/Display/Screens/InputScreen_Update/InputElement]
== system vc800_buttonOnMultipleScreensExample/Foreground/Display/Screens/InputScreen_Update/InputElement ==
  note: This Draw Button block shows the button on the screen. A button can only be drawn once per screen.
  In Bus Element{,1..17} (18 alike) : Inport
  function : TriggerPort  TriggerType=function-call  VariantControl=Variant
  Add1 : Sum
  Add2 : Sum
  Constant : Constant  Value=390  OutDataTypeStr=Inherit: Inherit via back propagation
  Constant1 : Constant  Value=20  OutDataTypeStr=int32
  Constant2 : Constant  Value=720  OutDataTypeStr=Inherit: Inherit via back propagation
  Constant25 : Constant  Value=200  OutDataTypeStr=int32
  Constant3 : Constant  Value=25  OutDataTypeStr=int32
  Constant4 : Constant  Value=20  OutDataTypeStr=int32
  Constant5 : Constant  Value=600  OutDataTypeStr=int32
  Data Type Conversion{,1..16} (17 alike) : DataTypeConversion
  Subsystem1 : Subsystem  mask{in_nam='Input9'}
      mask prompts: in_nam "Input Name"
  Subsystem10 : Subsystem  mask{in_nam='Input14'}
      mask prompts: in_nam "Input Name"
  Subsystem11 : Subsystem  mask{in_nam='Input13'}
      mask prompts: in_nam "Input Name"
  Subsystem12 : Subsystem  mask{in_nam='Input12'}
      mask prompts: in_nam "Input Name"
  Subsystem13 : Subsystem  mask{in_nam='Input11'}
      mask prompts: in_nam "Input Name"
  Subsystem14 : Subsystem  mask{in_nam='Input10'}
      mask prompts: in_nam "Input Name"
  Subsystem15 : Subsystem  mask{in_nam='Input15'}
      mask prompts: in_nam "Input Name"
  Subsystem16 : Subsystem  mask{in_nam='Input17'}
      mask prompts: in_nam "Input Name"
  Subsystem17 : Subsystem  mask{in_nam='Input16'}
      mask prompts: in_nam "Input Name"
  Subsystem18 : Subsystem  mask{in_nam='Input18'}
      mask prompts: in_nam "Input Name"
  Subsystem2 : Subsystem  mask{in_nam='Input8'}
      mask prompts: in_nam "Input Name"
  Subsystem3 : Subsystem  mask{in_nam='Input6'}
      mask prompts: in_nam "Input Name"
  Subsystem4 : Subsystem  mask{in_nam='Input5'}
      mask prompts: in_nam "Input Name"
  Subsystem5 : Subsystem  mask{in_nam='Input4'}
      mask prompts: in_nam "Input Name"
  Subsystem6 : Subsystem  mask{in_nam='Input3'}
      mask prompts: in_nam "Input Name"
  Subsystem7 : Subsystem  mask{in_nam='Input7'}
      mask prompts: in_nam "Input Name"
  Subsystem8 : Subsystem  mask{in_nam='Input1'}
      mask prompts: in_nam "Input Name"
  Subsystem9 : Subsystem  mask{in_nam='Input2'}
      mask prompts: in_nam "Input Name"
  Terminator : Terminator
  Terminator1 : Terminator
  display_draw_button : Raptor_display_lib/Drawing Functions/display_draw_button  ButtonName='GoToAbout'
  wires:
  In Bus Element1/1 -> Data Type Conversion/1
  In Bus Element2/1 -> Data Type Conversion1/1
  Constant1/1 -> Add1/2
  Add1/1 -> [XLeftCenter_Offset]
  Constant25/1 -> Add1/1, [XLeftCenter]
  In Bus Element3/1 -> Data Type Conversion2/1
  Data Type Conversion/1 -> Subsystem8/4(in_value)
  [XLeftCenter] -> Subsystem8/2(x)
  [XLeftCenter_Offset] -> Subsystem8/3(In3)
  Subsystem8/1(y_end_offset) -> Subsystem9/1(y_start_offset)
  Data Type Conversion1/1 -> Subsystem9/4(in_value)
  [XLeftCenter_Offset] -> Subsystem9/3(In3)
  [XLeftCenter] -> Subsystem9/2(x)
  [XLeftCenter] -> Subsystem6/2(x)
  [XLeftCenter_Offset] -> Subsystem6/3(In3)
  Data Type Conversion2/1 -> Subsystem6/4(in_value)
  Subsystem9/1(y_end_offset) -> Subsystem6/1(y_start_offset)
  Subsystem4/1(y_end_offset) -> Subsystem3/1(y_start_offset)
  Data Type Conversion5/1 -> Subsystem3/4(in_value)
  [XLeftCenter_Offset] -> Subsystem3/3(In3)
  [XLeftCenter] -> Subsystem3/2(x)
  [XLeftCenter] -> Subsystem4/2(x)
  [XLeftCenter_Offset] -> Subsystem4/3(In3)
  Data Type Conversion4/1 -> Subsystem4/4(in_value)
  Subsystem5/1(y_end_offset) -> Subsystem4/1(y_start_offset)
  [XLeftCenter_Offset] -> Subsystem5/3(In3)
  [XLeftCenter] -> Subsystem5/2(x)
  Data Type Conversion3/1 -> Subsystem5/4(in_value)
  Subsystem6/1(y_end_offset) -> Subsystem5/1(y_start_offset)
  In Bus Element4/1 -> Data Type Conversion3/1
  In Bus Element5/1 -> Data Type Conversion4/1
  In Bus Element6/1 -> Data Type Conversion5/1
  [XLeftCenter] -> Subsystem7/2(x)
  [XLeftCenter_Offset] -> Subsystem7/3(In3)
  Data Type Conversion6/1 -> Subsystem7/4(in_value)
  Subsystem3/1(y_end_offset) -> Subsystem7/1(y_start_offset)
  In Bus Element7/1 -> Data Type Conversion6/1
  [XRightCenter_Offset] -> Subsystem2/3(In3)
  [XRightCenter] -> Subsystem2/2(x)
  Data Type Conversion7/1 -> Subsystem2/4(in_value)
  Constant3/1 -> Subsystem8/1(y_start_offset), Subsystem2/1(y_start_offset)
  Constant5/1 -> [XRightCenter], Add2/1
  Add2/1 -> [XRightCenter_Offset]
  Constant4/1 -> Add2/2
  In Bus Element8/1 -> Data Type Conversion7/1
  In Bus Element9/1 -> Data Type Conversion8/1
  Data Type Conversion8/1 -> Subsystem1/4(in_value)
  [XRightCenter] -> Subsystem1/2(x)
  [XRightCenter_Offset] -> Subsystem1/3(In3)
  Subsystem2/1(y_end_offset) -> Subsystem1/1(y_start_offset)
  Subsystem1/1(y_end_offset) -> Subsystem14/1(y_start_offset)
  [XRightCenter_Offset] -> Subsystem14/3(In3)
  [XRightCenter] -> Subsystem14/2(x)
  Data Type Conversion9/1 -> Subsystem14/4(in_value)
  In Bus Element10/1 -> Data Type Conversion9/1
  In Bus Element11/1 -> Data Type Conversion10/1
  Data Type Conversion10/1 -> Subsystem13/4(in_value)
  [XRightCenter] -> Subsystem13/2(x)
  [XRightCenter_Offset] -> Subsystem13/3(In3)
  Subsystem14/1(y_end_offset) -> Subsystem13/1(y_start_offset)
  Subsystem13/1(y_end_offset) -> Subsystem12/1(y_start_offset)
  [XRightCenter_Offset] -> Subsystem12/3(In3)
  [XRightCenter] -> Subsystem12/2(x)
  Data Type Conversion11/1 -> Subsystem12/4(in_value)
  Data Type Conversion12/1 -> Subsystem11/4(in_value)
  [XRightCenter] -> Subsystem11/2(x)
  [XRightCenter_Offset] -> Subsystem11/3(In3)
  Subsystem12/1(y_end_offset) -> Subsystem11/1(y_start_offset)
  Subsystem11/1(y_end_offset) -> Subsystem10/1(y_start_offset)
  [XRightCenter_Offset] -> Subsystem10/3(In3)
  [XRightCenter] -> Subsystem10/2(x)
  Data Type Conversion13/1 -> Subsystem10/4(in_value)
  In Bus Element12/1 -> Data Type Conversion11/1
  In Bus Element13/1 -> Data Type Conversion12/1
  In Bus Element14/1 -> Data Type Conversion13/1
  In Bus Element/1 -> Data Type Conversion14/1
  Subsystem7/1(y_end_offset) -> Subsystem15/1(y_start_offset)
  [XLeftCenter] -> Subsystem15/2(x)
  [XLeftCenter_Offset] -> Subsystem15/3(x1)
  Data Type Conversion14/1 -> Subsystem15/4(in_value)
  Data Type Conversion15/1 -> Subsystem16/4(in_value)
  [XLeftCenter_Offset] -> Subsystem16/3(x1)
  [XLeftCenter] -> Subsystem16/2(x)
  Subsystem15/1(y_end_offset) -> Subsystem16/1(y_start_offset)
  In Bus Element16/1 -> Data Type Conversion15/1
  Data Type Conversion16/1 -> Subsystem17/4(in_value)
  [XRightCenter_Offset] -> Subsystem17/3(x1)
  [XRightCenter] -> Subsystem17/2(x)
  Subsystem10/1(y_end_offset) -> Subsystem17/1(y_start_offset)
  In Bus Element15/1 -> Data Type Conversion16/1
  Subsystem16/1(y_end_offset) -> Terminator/1
  Subsystem17/1(y_end_offset) -> Subsystem18/1(y_start_offset)
  In Bus Element17/1 -> Subsystem18/4(in_value)
  [XRightCenter] -> Subsystem18/2(x)
  [XRightCenter_Offset] -> Subsystem18/3(In3)
  Subsystem18/1(y_end_offset) -> Terminator1/1
  Constant2/1 -> display_draw_button/1
  Constant/1 -> display_draw_button/2

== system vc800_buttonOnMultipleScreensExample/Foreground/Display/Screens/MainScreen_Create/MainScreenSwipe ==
  note: This function is called when a swipe action occurs. The gesture input will provide the gesture detected: 0 = UP 1 = DOWN 2 = LEFT 3 = RIGHT
  MainScreenSwipe : TriggerPort  TriggerType=function-call  IsSimulinkFunction=on  FunctionName=MainScreenSwipe  FunctionVisibility=scoped  VariantControl=Variant  PortDimensions=1
  Constant : Constant  OutDataTypeStr=uint8
  Function Caller : FunctionCaller  FunctionPrototype=Screens.Navigation(gesture,curr_screen)  InputArgumentSpecifications=<Enter example>  OutputArgumentSpecifications=<Enter example>
  gesture : ArgIn  OutDataTypeStr=uint8  ArgumentName=gesture
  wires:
  gesture/1 -> Function Caller/1
  Constant/1 -> Function Caller/2

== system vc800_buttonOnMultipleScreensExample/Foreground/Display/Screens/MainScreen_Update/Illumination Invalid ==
  Xbase : Inport
  Ybase : Inport  Port=2
  Prev : Inport  Port=3
  Enable : EnablePort
  Add : Sum
  Add1 : Sum  Inputs=+-
  Constant1 : Constant  Value=51  OutDataTypeStr=int32
  Constant74 : Constant  Value=20  OutDataTypeStr=int32
  Terminator : Terminator
  display_draw_image : Raptor_display_lib/Drawing Functions/display_draw_image  imagePort=off  imageFile=FaultRED.bmp  opacityPort=off  opacity=100  drawMode=Draw Entire Image  alpha=Draw as Transparent  layer=Background  drawModeXY=Top Left  pnPort=on
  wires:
  display_draw_image/1 -> Terminator/1
  Prev/1 -> display_draw_image/1
  Add/1 -> display_draw_image/3
  Constant74/1 -> Add/2
  Ybase/1 -> Add/1
  Constant1/1 -> Add1/2
  Xbase/1 -> Add1/1
  Add1/1 -> display_draw_image/2

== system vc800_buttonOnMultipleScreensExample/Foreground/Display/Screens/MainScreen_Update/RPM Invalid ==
  Xbase : Inport
  Ybase : Inport  Port=2
  Prev : Inport  Port=3
  Enable : EnablePort
  Add : Sum
  Constant74 : Constant  Value=20  OutDataTypeStr=int32
  Terminator : Terminator
  display_draw_image : Raptor_display_lib/Drawing Functions/display_draw_image  imagePort=off  imageFile=FaultRED.bmp  opacityPort=off  opacity=100  drawMode=Draw Entire Image  alpha=Draw as Transparent  layer=Background  drawModeXY=Top Left  pnPort=on
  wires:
  Xbase/1 -> display_draw_image/2
  Ybase/1 -> Add/1
  Constant74/1 -> Add/2
  Add/1 -> display_draw_image/3
  Prev/1 -> display_draw_image/1
  display_draw_image/1 -> Terminator/1

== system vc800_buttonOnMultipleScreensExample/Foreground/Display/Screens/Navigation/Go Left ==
  Current Screen : Inport
  Action Port : ActionPort  ActionPortLabel=elseif(u1 == 2)
  About : Subsystem  TreatAsAtomicUnit=on
  DataLog : Subsystem  TreatAsAtomicUnit=on
  Default : Subsystem  TreatAsAtomicUnit=on
  Input : Subsystem  TreatAsAtomicUnit=on
  Main : Subsystem  TreatAsAtomicUnit=on
  Output : Subsystem  TreatAsAtomicUnit=on
  Switch Case1 : SwitchCase  CaseConditions={1,2,3,4,5}
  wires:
  Switch Case1/2 -> Input/Action
  Switch Case1/6 -> Default/Action
  Switch Case1/5 -> About/Action
  Switch Case1/1 -> Main/Action
  Switch Case1/4 -> DataLog/Action
  Current Screen/1 -> Switch Case1/1
  Switch Case1/3 -> Output/Action
